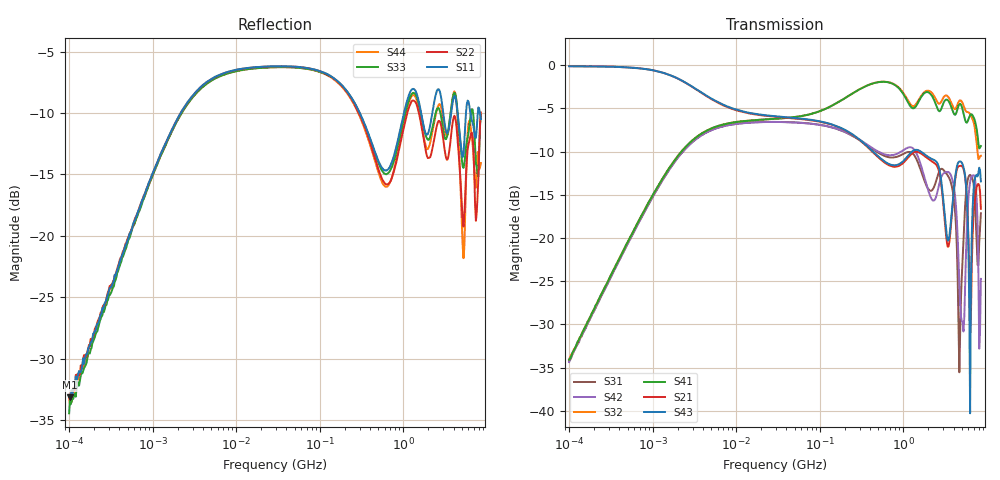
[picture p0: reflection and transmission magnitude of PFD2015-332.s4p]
# MHz S MA R 50
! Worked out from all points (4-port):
!   498 points, 100 kHz to 8.5 GHz, reference 50 ohm
!   strongest paths, dB at 100 kHz, 1.698 MHz, 29.49 MHz, 500.7 MHz, 8.5 GHz:
!     S43: -0.1, -1.2, -5.9, -10.5, -13.4
!     S21: -0.1, -1.2, -6.0, -10.6, -16.6
!     S41: -34.1, -11.5, -6.2, -2.0, -9.4
!     S32: -34.0, -11.5, -6.2, -2.0, -10.5
!     S42: -34.4, -11.7, -6.6, -10.0, -24.7
!     S31: -34.2, -11.6, -6.6, -10.1, -17.1
!   lowest |S11| = -33.1 dB at 102.3 kHz (marker M1), VSWR 1.05, Z = 51 + j2.01 ohm
!   |S11| at or under -10 dB: 302.3 MHz to 1.02 GHz (717.3 MHz wide, 109 % of centre); 4.47 GHz to 5.633 GHz (1.163 GHz wide, 23 % of centre); 6.359 GHz to 7.816 GHz (1.457 GHz wide, 20.6 % of centre)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
0.1  0.02233 63.7  0.986 -1.1  0.01942 -93.3  0.01977 85.7
     0.986 -1.1  0.02215 69.3  0.01986 86.9  0.01915 -93.9
     0.01942 -93.3  0.01986 86.9  0.01897 60.5  0.9853 -1.1
     0.01977 85.7  0.01915 -93.9  0.9853 -1.1  0.02185 66.6
0.1023101  0.02202 63.5  0.9861 -1.2  0.01962 -93.6  0.02013 86.3
           0.9861 -1.2  0.02263 70.2  0.02036 85.9  0.02014 -93.9
           0.01962 -93.6  0.02036 85.9  0.02151 62.6  0.9846 -1.2
           0.02013 86.3  0.02014 -93.9  0.9846 -1.2  0.02059 64.7
10.08106  0.4747 11.7  0.5478 -16.2  0.4575 -169.5  0.469 14.5
          0.5478 -16.2  0.4741 11.5  0.4693 14.5  0.457 -169.6
          0.4575 -169.5  0.4693 14.5  0.4682 11.9  0.5529 -16.2
          0.469 14.5  0.457 -169.6  0.5529 -16.2  0.4684 11.8
658.5124  0.1868 -85.6  0.265 173.6  0.2938 -5.3  0.7961 -88.2
          0.265 173.6  0.1622 -88.8  0.7978 -87.4  0.3018 -9.4
          0.2938 -5.3  0.7978 -87.4  0.18 -87.3  0.2694 173.1
          0.7961 -88.2  0.3018 -9.4  0.2694 173.1  0.1603 -87.0
1498.389  0.3651 148.4  0.3143 -59.3  0.2736 131.0  0.6045 168.0
          0.3143 -59.3  0.3285 148.0  0.6181 168.4  0.2953 134.3
          0.2736 131.0  0.6181 168.4  0.355 145.9  0.3229 -60.3
          0.6045 168.0  0.2953 134.3  0.3229 -60.3  0.344 147.1
2652.059  0.3954 18.3  0.2476 29.1  0.2379 173.4  0.5448 9.8
          0.2476 29.1  0.2937 24.5  0.5986 11.1  0.1979 -177.8
          0.2379 173.4  0.5986 11.1  0.3315 12.7  0.2596 26.5
          0.5448 9.8  0.1979 -177.8  0.2596 26.5  0.3419 22.1
8500  0.2988 -50.8  0.1475 2.7  0.1391 60.4  0.3403 -29.0
      0.1475 2.7  0.3181 -31.8  0.2988 -29.7  0.05803 64.1
      0.1391 60.4  0.2988 -29.7  0.3111 -37.4  0.2126 6.9
      0.3403 -29.0  0.05803 64.1  0.2126 6.9  0.198 -32.6
